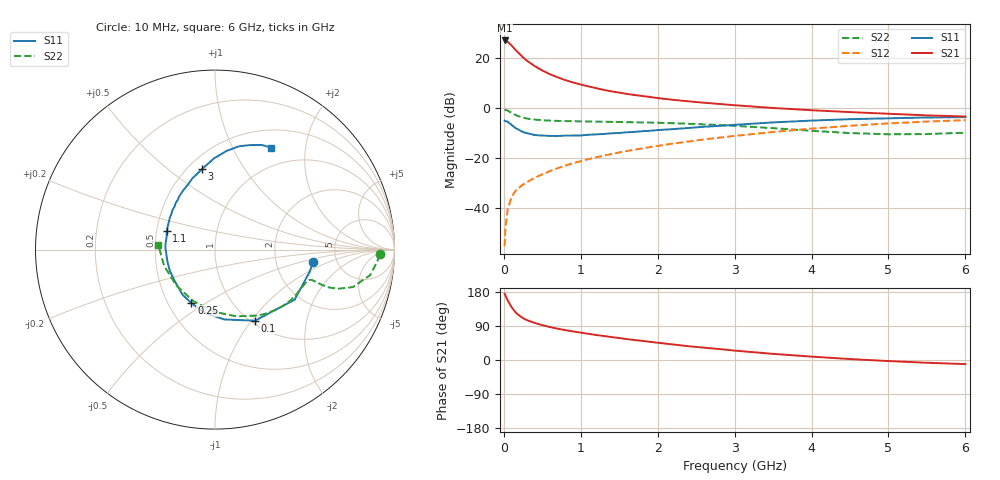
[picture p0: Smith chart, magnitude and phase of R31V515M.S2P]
! SIEMENS Small Signal Semiconductors
! BFR181
! Si NPN RF Bipolar Junction Transistor in SOT23
! VCE = 1.5 V  IC = 15 mA
! Common Emitter S-Parameters:  May  1996
# GHz  S  MA  R  50
!  f  S11  S21  S12  S22
! GHz  MAG  ANG  MAG  ANG  MAG  ANG  MAG  ANG
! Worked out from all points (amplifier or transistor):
!   36 points, 10 MHz to 6 GHz, reference 50 ohm
!   highest |S21| = 26.9 dB at 10 MHz (marker M1)
!   |S21| within 3 dB of that: start of sweep to 129.2 MHz
!   unconditionally stable (mu >= 1): start of sweep to 14.87 MHz; 291.1 MHz to 3.664 GHz; 5.681 GHz to end of sweep
!   at 250 MHz: K = 0.93, MSG = 25.4 dB, |S12| = -30.7 dB
!   at 1.4 GHz: K = 1.28, MAG = 9.4 dB, |S12| = -18.5 dB
!   at 6 GHz: K = 1.01, MAG = 0.1 dB, |S12| = -5.0 dB
!   S11 on the Smith chart (normalised r, x): 10 MHz: 3.31, -0.66; 100 MHz: 1.04, -1.04; 250 MHz: 0.65, -0.43; 1.1 GHz: 0.57, +0.13; 3 GHz: 0.59, +0.67; 6 GHz: 0.73, +1.43
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0.01  0.5508 -7.2  22.19 175.1  0.0017 85.8  0.917 -1.7
0.02  0.5416 -13.3  21.93 170.4  0.0039 83.0  0.9076 -4.0
0.05  0.524 -32.2  20.85 157.5  0.0093 75.9  0.8765 -9.3
0.1  0.4545 -60.6  17.63 139.7  0.0164 68.6  0.7962 -15.2
0.15  0.3927 -82.4  14.47 126.2  0.0216 64.0  0.7182 -17.7
0.2  0.3583 -99.2  12.08 117.3  0.0253 64.3  0.6678 -18.4
0.25  0.3256 -113.9  10.14 110.4  0.0292 63.7  0.6332 -18.3
0.3  0.3098 -125.7  8.733 105.2  0.0325 65.2  0.6078 -18.0
0.4  0.2843 -142.5  6.832 98.0  0.0396 66.6  0.5799 -17.6
0.5  0.2777 -155.7  5.55 91.8  0.0465 68.8  0.5637 -17.4
0.6  0.2732 -166.3  4.673 86.9  0.0541 70.0  0.5527 -17.8
0.8  0.2772 177.5  3.567 78.8  0.0695 70.9  0.5407 -19.3
0.9  0.2776 171.4  3.203 75.3  0.0778 71.4  0.5371 -20.2
1.1  0.2876 159.1  2.673 69.1  0.0936 72.1  0.5305 -22.7
1.3  0.2987 149.8  2.274 63.3  0.1103 71.7  0.5246 -25.2
1.6  0.3231 137.3  1.887 55.1  0.1364 70.6  0.515 -29.8
2.2  0.3738 118.4  1.44 41.0  0.192 67.2  0.4897 -40.3
3  0.4549 99.1  1.122 24.8  0.2733 59.9  0.4348 -57.7
3.5  0.5091 90.5  0.989 16.2  0.3275 54.2  0.3901 -72.4
4.5  0.5906 77.0  0.818 2.5  0.4356 40.8  0.3115 -112.8
5.5  0.638 66.0  0.703 -7.3  0.5289 25.7  0.2975 -162.2
6  0.6497 61.1  0.668 -10.8  0.5644 18.0  0.3168 175.5
